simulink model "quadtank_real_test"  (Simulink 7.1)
settings: Solver=ode45  StartTime=0.0  StopTime=150  RelTol=1e-6
PreLoadFcn:
  | init_quadtank
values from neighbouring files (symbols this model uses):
  W1 = eye(2)    [init_quadtank.m]
  W2 = eye(2)    [init_quadtank.m]
libraries: cstblocks x2

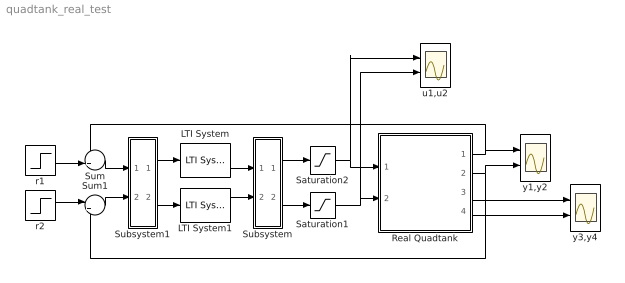
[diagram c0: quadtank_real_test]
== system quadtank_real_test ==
  LTI System : cstblocks/LTI System  SystemSampleTime=-1  sys=C1  IC=[]
  LTI System1 : cstblocks/LTI System  SystemSampleTime=-1  sys=C2  IC=[]
  Real Quadtank : Subsystem  AncestorBlock=tank/Real Quadtank  mask{h=0.05}
  Saturation1 : Saturate  UpperLimit=10  LowerLimit=0
  Saturation2 : Saturate  UpperLimit=10  LowerLimit=0
  Subsystem : Subsystem
  Subsystem1 : Subsystem
  Sum : Sum  Inputs=-+|
  Sum1 : Sum  Inputs=|+-
  r1 : Step  Time=50  Before=5  After=6  SampleTime=0
  r2 : Step  Time=100  Before=5  After=6  SampleTime=0
  u1,u2 : Scope  NumInputPorts=2
  y1,y2 : Scope  NumInputPorts=2
  y3,y4 : Scope  NumInputPorts=2
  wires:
  Real Quadtank/1(y1) -> Sum/1, y1,y2/1
  Real Quadtank/2(y2) -> Sum1/2, y1,y2/2
  r2/1 -> Sum1/1
  Real Quadtank/3(y3) -> y3,y4/1
  Real Quadtank/4(y4) -> y3,y4/2
  Saturation2/1 -> u1,u2/1, Real Quadtank/1(u1)
  Saturation1/1 -> u1,u2/2, Real Quadtank/2(u2)
  LTI System/1 -> Subsystem/1(In1)
  LTI System1/1 -> Subsystem/2(In2)
  Subsystem1/1(Out1) -> LTI System/1
  Subsystem1/2(Out2) -> LTI System1/1
  Subsystem/1(Out1) -> Saturation2/1
  Subsystem/2(Out2) -> Saturation1/1
  Sum/1 -> Subsystem1/1(In1)
  Sum1/1 -> Subsystem1/2(In2)
  r1/1 -> Sum/2

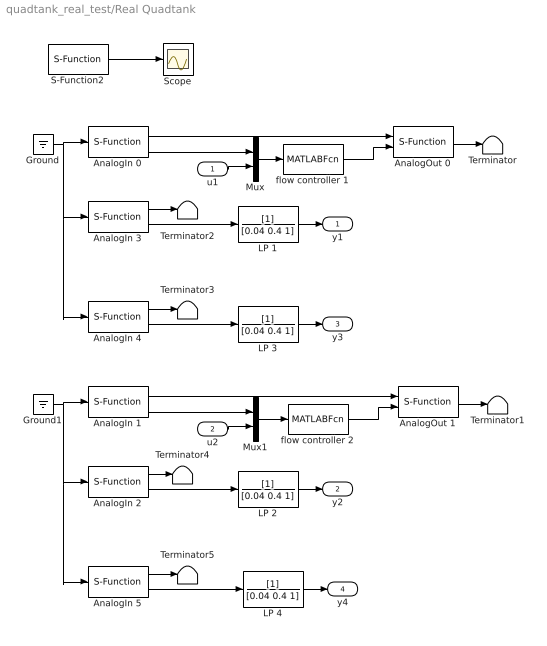
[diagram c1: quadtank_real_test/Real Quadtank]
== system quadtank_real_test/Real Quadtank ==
  u1 : Inport  OutDataType=sfix(16)  OutScaling=2^0
  u2 : Inport  Port=2  OutDataType=sfix(16)  OutScaling=2^0
  AnalogIn 0 : S-Function  FunctionName=analogin  Parameters=h [35]  EnableBusSupport=off
  AnalogIn 1 : S-Function  FunctionName=analogin  Parameters=h [34]  EnableBusSupport=off
  AnalogIn 2 : S-Function  FunctionName=analogin  Parameters=h [33]  EnableBusSupport=off
  AnalogIn 3 : S-Function  FunctionName=analogin  Parameters=h [31]  EnableBusSupport=off
  AnalogIn 4 : S-Function  FunctionName=analogin  Parameters=h [30]  EnableBusSupport=off
  AnalogIn 5 : S-Function  FunctionName=analogin  Parameters=h [32]  EnableBusSupport=off
  AnalogOut 0 : S-Function  FunctionName=analogout  Parameters=h [31]  EnableBusSupport=off
  AnalogOut 1 : S-Function  FunctionName=analogout  Parameters=h [30]  EnableBusSupport=off
  Ground : Ground
  Ground1 : Ground
  LP {1..4} (4 alike) : TransferFcn  Denominator=[0.04 0.4 1]
  Mux : Mux  Inputs=2
  Mux1 : Mux  Inputs=2
  S-Function2 : S-Function  FunctionName=realtimer  Parameters=h  EnableBusSupport=off
  Scope : Scope
  Terminator{,1..5} (6 alike) : Terminator
  flow controller 1 : MATLABFcn  MATLABFcn=flowCtrl1  SampleTime=0.01
  flow controller 2 : MATLABFcn  MATLABFcn=flowCtrl2  SampleTime=0.01
  y1 : Outport  OutDataType=sfix(16)  OutScaling=2^0
  y2 : Outport  Port=2  OutDataType=sfix(16)  OutScaling=2^0
  y3 : Outport  Port=3  OutDataType=sfix(16)  OutScaling=2^0
  y4 : Outport  Port=4  OutDataType=sfix(16)  OutScaling=2^0
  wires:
  S-Function2/1 -> Scope/1
  AnalogIn 0/1 -> AnalogOut 0/1
  AnalogOut 0/1 -> Terminator/1
  AnalogIn 1/1 -> AnalogOut 1/1
  AnalogOut 1/1 -> Terminator1/1
  AnalogIn 3/2 -> LP 1/1
  AnalogIn 4/2 -> LP 3/1
  Ground/1 -> AnalogIn 0/1, AnalogIn 3/1, AnalogIn 4/1
  AnalogIn 3/1 -> Terminator2/1
  AnalogIn 4/1 -> Terminator3/1
  AnalogIn 2/2 -> LP 2/1
  AnalogIn 5/2 -> LP 4/1
  Ground1/1 -> AnalogIn 5/1, AnalogIn 2/1, AnalogIn 1/1
  AnalogIn 2/1 -> Terminator4/1
  AnalogIn 5/1 -> Terminator5/1
  u1/1 -> Mux/2
  Mux/1 -> flow controller 1/1
  flow controller 1/1 -> AnalogOut 0/2
  u2/1 -> Mux1/2
  Mux1/1 -> flow controller 2/1
  flow controller 2/1 -> AnalogOut 1/2
  AnalogIn 1/2 -> Mux1/1
  AnalogIn 0/2 -> Mux/1
  LP 1/1 -> y1/1
  LP 3/1 -> y3/1
  LP 2/1 -> y2/1
  LP 4/1 -> y4/1

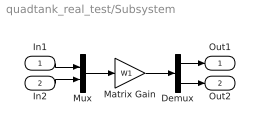
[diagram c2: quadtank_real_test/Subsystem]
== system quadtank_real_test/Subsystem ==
  In1 : Inport
  In2 : Inport  Port=2
  Demux : Demux  Outputs=2
  Matrix Gain : Gain  Gain=W1  Multiplication=Matrix(K*u)
  Mux : Mux  Inputs=2
  Out1 : Outport
  Out2 : Outport  Port=2
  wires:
  Demux/1 -> Out1/1
  In1/1 -> Mux/1
  Demux/2 -> Out2/1
  In2/1 -> Mux/2
  Mux/1 -> Matrix Gain/1
  Matrix Gain/1 -> Demux/1

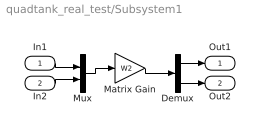
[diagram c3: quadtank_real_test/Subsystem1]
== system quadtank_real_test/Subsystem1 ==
  In1 : Inport
  In2 : Inport  Port=2
  Demux : Demux  Outputs=2
  Matrix Gain : Gain  Gain=W2  Multiplication=Matrix(K*u)
  Mux : Mux  Inputs=2
  Out1 : Outport
  Out2 : Outport  Port=2
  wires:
  Matrix Gain/1 -> Demux/1
  Mux/1 -> Matrix Gain/1
  In2/1 -> Mux/2
  Demux/2 -> Out2/1
  In1/1 -> Mux/1
  Demux/1 -> Out1/1
